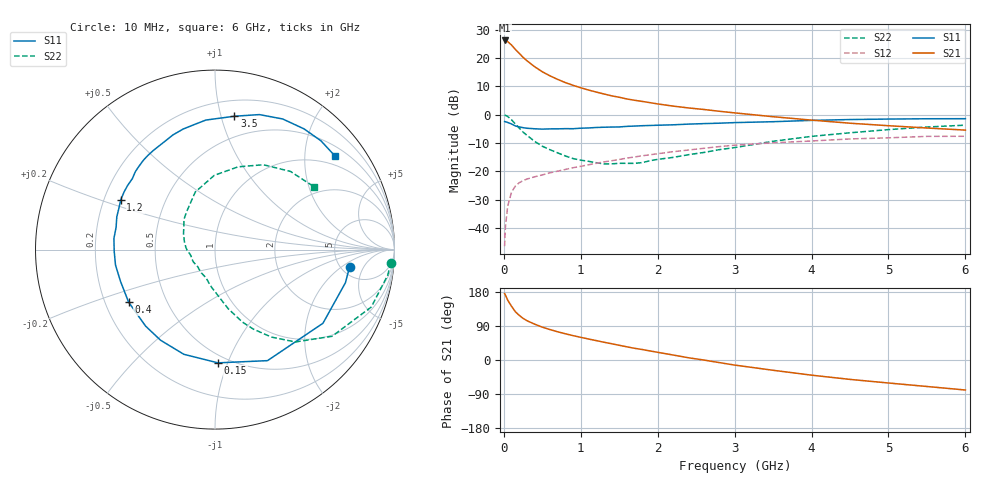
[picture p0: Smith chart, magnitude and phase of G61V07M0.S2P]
! SIEMENS Small Signal Semiconductors
! BFG193
! Si NPN RF Bipolar Junction Transistor in SOT223
! VCE = 1 V  IC = 7 mA
! Common Emitter S-Parameters:  August  1996
# GHz  S  MA  R  50
!  f  S11  S21  S12  S22
! GHz  MAG  ANG  MAG  ANG  MAG  ANG  MAG  ANG
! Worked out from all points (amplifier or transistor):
!   36 points, 10 MHz to 6 GHz, reference 50 ohm
!   highest |S21| = 26.2 dB at 10 MHz (marker M1)
!   |S21| within 3 dB of that: start of sweep to 144.8 MHz
!   unconditionally stable (mu >= 1): 944.4 MHz to 3.156 GHz
!   at 250 MHz: K = 0.43, MSG = 21.7 dB, |S12| = -23.3 dB
!   at 1.4 GHz: K = 1.09, MAG = 9.6 dB, |S12| = -16.3 dB
!   at 6 GHz: K = 0.96, MSG = 1.1 dB, |S12| = -7.6 dB
!   S11 on the Smith chart (normalised r, x): 10 MHz: 5.97, -2.67; 150 MHz: 0.44, -0.92; 400 MHz: 0.30, -0.26; 1.2 GHz: 0.27, +0.23; 3.5 GHz: 0.32, +1.10; 6 GHz: 0.74, +2.74
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0.01  0.7559 -7.3  20.31 175.3  0.0048 90.7  0.9825 -4.2
0.02  0.7499 -14.2  20.21 171.8  0.0103 84.6  0.9731 -8.4
0.05  0.7282 -34.3  19.34 158.0  0.0245 73.2  0.9275 -20.2
0.1  0.6843 -64.7  16.87 141.7  0.0431 61.0  0.8117 -36.5
0.15  0.6312 -88.5  14.12 127.3  0.0551 51.5  0.6819 -49.0
0.2  0.6086 -106.6  12.04 117.8  0.063 46.7  0.5797 -57.2
0.25  0.589 -121.0  10.25 109.9  0.0686 43.3  0.4925 -64.2
0.3  0.5755 -132.2  8.917 103.8  0.0732 41.3  0.4326 -69.2
0.4  0.5634 -148.7  7.004 94.6  0.0801 39.5  0.3384 -77.3
0.5  0.5554 -161.6  5.697 86.7  0.0866 38.6  0.2777 -83.4
0.6  0.561 -171.2  4.83 80.3  0.0943 38.7  0.2405 -88.9
0.7  0.5617 -179.1  4.182 74.4  0.1009 38.8  0.2119 -94.9
0.9  0.5647 167.4  3.289 64.3  0.116 39.1  0.1681 -106.4
1.1  0.5824 157.0  2.714 55.4  0.1306 38.2  0.1505 -120.3
1.2  0.5938 152.2  2.504 51.3  0.1385 37.8  0.1422 -127.6
1.6  0.6209 135.6  1.889 34.7  0.1713 33.5  0.1386 -157.1
2.2  0.6619 115.9  1.414 13.2  0.2221 24.1  0.1763 165.3
2.8  0.7067 99.2  1.147 -6.8  0.2732 12.6  0.2412 135.9
3.5  0.7509 81.7  0.919 -27.1  0.319 -3.5  0.3392 108.9
4.5  0.8197 62.6  0.706 -51.2  0.373 -22.6  0.4788 74.4
5.5  0.8461 45.8  0.581 -69.9  0.4138 -45.6  0.6054 46.0
6  0.8481 37.8  0.534 -79.2  0.4156 -58.8  0.6525 32.6
